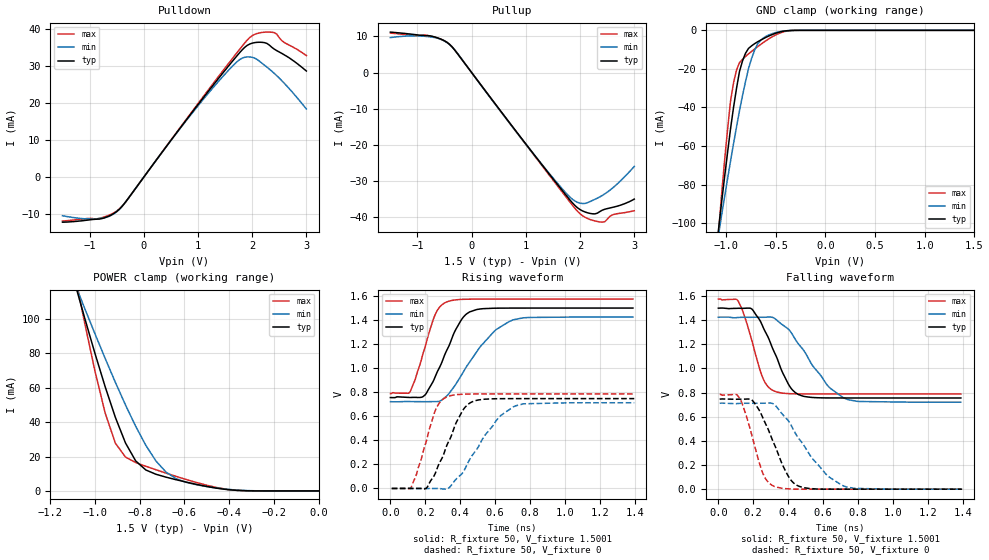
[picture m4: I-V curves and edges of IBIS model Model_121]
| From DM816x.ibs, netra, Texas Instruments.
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| Model based on original model for BSHTLTCSCDVGPBFZ
|   Sub model SLOWEST_8MA_5PER_1P5
[model]   Model_121
|[Description]  1.5V-3-STATE-X-SLOWEST, 8MA, +-5%
|[Input Load]
|[Output Drive] SLOWEST, 8MA
|Voltage   1.5V
|Mode   3-STATE
Model_type   3-state
Polarity   Non-Inverting
Enable   Active-Low
Cref =  15.0000pF
Rref =  100.0000M
Vref =  0V
Vmeas =  0.75005
C_comp   1.5249p   1.4275p   1.6205p
[Model Spec]
[Temperature Range]   25   125   -40
[Voltage Range]   1.5   1.425   1.575
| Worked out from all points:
|   slope of the pulldown table from 0 to 0.225 V, typ, clamps not added: 50.1 ohm
|   slope of the pullup table from 0 to 0.225 V, typ, clamps not added: 50.1 ohm
|   GND clamp passes 1 mA (typ) near -0.47 V on its own axis
|   POWER clamp passes 1 mA (typ) near -0.42 V on its own axis
|   rising waveform, R_fixture 50, V_fixture 1.5001: 20-80 % time 136ps typ, 208ps min, 98.4ps max; typ from 0.756 V to 1.5 V
|   rising waveform, R_fixture 50, V_fixture 0: 20-80 % time 132ps typ, 190ps min, 95.5ps max; typ from 0 V to 0.747 V
|   falling waveform, R_fixture 50, V_fixture 1.5001: 20-80 % time 135ps typ, 201ps min, 94.8ps max; typ from 1.5 V to 0.755 V
|   falling waveform, R_fixture 50, V_fixture 0: 20-80 % time 132ps typ, 207ps min, 92.6ps max; typ from 0.746 V to 0 V
[POWER_clamp]
-1.5V     321.7mA    260.6mA    415.9mA
-1.076V   114.2mA    115.8mA    116.9mA
-1.061V   107.2mA    110.9mA    107.1mA
-954.6mV  60.59mA    77.06mA    45.35mA
-909.2mV  42.85mA    63.21mA    27.81mA
-863.7mV  27.9mA     49.99mA    19.69mA
-818.2mV  17.49mA    37.63mA    16.52mA
-772.8mV  12.19mA    26.53mA    14.33mA
-681.9mV  7.985mA    10.89mA    10.33mA
-590.9mV  5.094mA    4.955mA    6.6mA
-363.7mV  298.5uA    465.2uA    297.6uA
0V        1.518nA    24.08nA    367.8pA
[Pulldown]
-1.5V     -12.15mA   -10.4mA    -11.83mA
-863.7mV  -11.34mA   -11.22mA   -11.25mA
-500mV    -9.267mA   -9.352mA   -9.148mA
-318.2mV  -6.354mA   -6.371mA   -6.385mA
1.046V    20.42mA    20.05mA    20.72mA
1.591V    30.47mA    29.26mA    31.18mA
1.818V    34.39mA    32.13mA    35.4mA
1.955V    35.92mA    32.45mA    37.67mA
2.091V    36.38mA    31.76mA    38.77mA
2.273V    36.08mA    29.69mA    39.15mA
2.364V    35.03mA    28.59mA    39.11mA
3V        28.64mA    18.41mA    32.82mA
[Pullup]
-1.5V     11.21mA    9.69mA     10.94mA
-818.2mV  10.23mA    9.978mA    10.29mA
-590.9mV  9.401mA    9.328mA    9.374mA
-409.1mV  7.828mA    7.781mA    7.859mA
1.227V    -24.14mA   -24.11mA   -24.35mA
1.727V    -33.63mA   -33.09mA   -34.13mA
1.909V    -36.81mA   -35.55mA   -37.6mA
2.046V    -38.25mA   -36.2mA    -39.57mA
2.227V    -39.04mA   -35.36mA   -40.83mA
2.409V    -38.05mA   -33.98mA   -41.36mA
2.591V    -37.29mA   -32.03mA   -39.38mA
3V        -34.98mA   -25.95mA   -38.2mA
[GND_clamp]
-1.5V     -310.1mA   -250.5mA   -402.5mA
-1.076V   -103.6mA   -106.2mA   -105.2mA
-1.046V   -89.81mA   -96.36mA   -86.02mA
-954.6mV  -51.22mA   -67.87mA   -36.88mA
-924.3mV  -40.08mA   -58.86mA   -27.29mA
-863.7mV  -21.24mA   -41.56mA   -16.73mA
-833.4mV  -15.8mA    -33.75mA   -15.03mA
-772.8mV  -9.345mA   -19.75mA   -12.19mA
-712.2mV  -6.928mA   -10.35mA   -9.704mA
-621.3mV  -4.261mA   -3.896mA   -6.225mA
-409.1mV  -337.1uA   -289.1uA   -618.9uA
1.5V      1.518nA    257.2nA    299pA
[Ramp]
dV/dt_f   0.596016/0.19469535n   0.56432/0.3101823n   0.629272/0.14102085n
dV/dt_r  0.6013584/0.19239092n 0.57508648/0.29752883n 0.63081544/0.1406002n
R_load = 50
[Rising Waveform]
R_fixture = 50
V_fixture = 1.5001
V_fixture_min = 1.425
V_fixture_max = 1.575
0s        755.9mV    721.6mV    789.3mV
113.1ps   756.8mV    722.8mV    805.9mV
202.4ps   784.3mV    721.6mV    1.194V
258.2ps   935mV      722.2mV    1.452V
322.4ps   1.148V     768.9mV    1.551V
401.7ps   1.391V     930.2mV    1.572V
453.8ps   1.468V     1.051V     1.574V
593.7ps   1.499V     1.306V     1.575V
703.7ps   1.5V       1.403V     1.575V
1.389ns   1.5V       1.425V     1.575V
[Rising Waveform]
R_fixture = 50
V_fixture = 0
V_fixture_min = 0
V_fixture_max = 0
7.64ps    0V         0V         0V
115.8ps   0V         2.005mV    0V
205.8ps   0V         0V         393mV
264.7ps   154.4mV    0V         672.8mV
328.5ps   375.7mV    0V         764.9mV
407.5ps   630.7mV    119.4mV    783.3mV
453.4ps   709mV      239.6mV    785.2mV
616.4ps   746.3mV    583.8mV    786.2mV
716.3ps   747.1mV    687mV      786.3mV
1.397ns   747.3mV    712.8mV    786.3mV
[Falling Waveform]
R_fixture = 50
V_fixture = 1.5001
V_fixture_min = 1.425
V_fixture_max = 1.575
0s        1.499V     1.424V     1.575V
112.8ps   1.498V     1.422V     1.559V
196.7ps   1.485V     1.424V     1.207V
258.2ps   1.336V     1.424V     910.4mV
319.4ps   1.139V     1.417V     813mV
398.9ps   876.3mV    1.329V     791.5mV
443.3ps   797.6mV    1.235V     789.6mV
622ps     755.7mV    865.1mV    788.6mV
724ps     755.3mV    752mV      788.6mV
1.389ns   755.2mV    720.6mV    788.5mV
[Falling Waveform]
R_fixture = 50
V_fixture = 0
V_fixture_min = 0
V_fixture_max = 0
7.64ps    746.3mV    712.1mV    785.4mV
121.1ps   745.4mV    710.4mV    755.3mV
189.6ps   741.3mV    711.4mV    460.1mV
252.7ps   598.9mV    711.6mV    139.8mV
322.1ps   366.5mV    698.9mV    21.87mV
396.8ps   117.8mV    574.2mV    3.273mV
443.5ps   37.83mV    457.1mV    0V
617.3ps   0V         122.8mV    0V
715.1ps   0V         28.16mV    0V
1.397ns   0V         0V         0V
